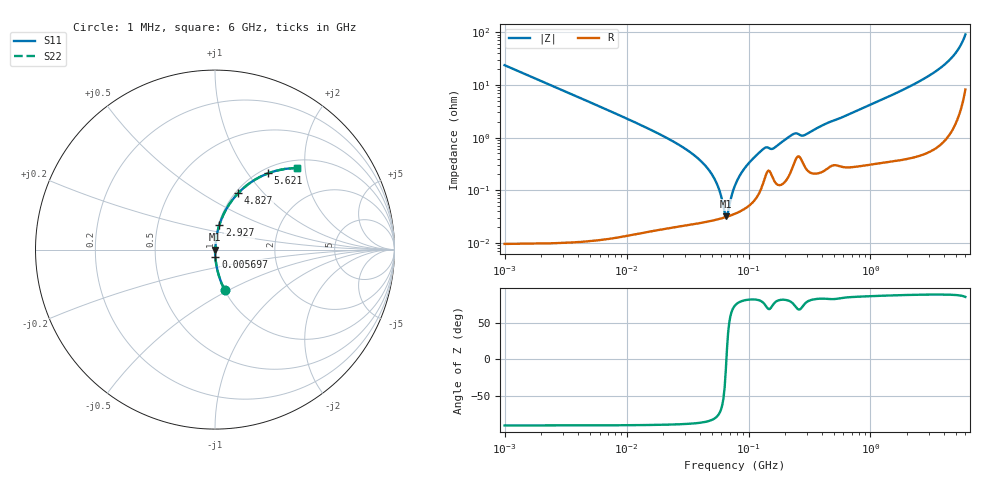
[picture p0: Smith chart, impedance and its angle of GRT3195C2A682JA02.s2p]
!Murata Part Number: GRT3195C2A682JA02
!These Parameters are Measured in Series Mode Connection
!Data Generated on Jun 19, 2026
!  o--ll--o
!Port1  Port2
!  o------o
!Operation Temp=25[degC], DC Bias Voltage=0[V]
!Freq. Start=1000[kHz] Stop=6[GHz] 401[Steps]
# Hz S RI R 50
!Freq.(Hz) S11(Real) S11(Imag) S21(Real) S21(Imag) S12(Real) S12(Imag) S22(Real) S22(Imag)
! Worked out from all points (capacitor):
!   401 points, 1 MHz to 6 GHz, reference 50 ohm
!   read as one part in series: C = 6.73 nF near 1.044 MHz
!   lowest |Z| = 32.2 mohm at 65.09 MHz (marker M1)
!   series resonance near 65.87 MHz, so ESL is about 870 pH
!   S11 on the Smith chart (normalised r, x): 1 MHz: 1.00, -0.47; 5.697 MHz: 1.00, -0.08; 2.927 GHz: 1.01, +0.29; 4.827 GHz: 1.03, +0.73; 5.621 GHz: 1.08, +1.25; 6 GHz: 1.16, +1.80
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1000000  0.053 -0.2238  0.947 0.2238  0.947 0.2238  0.053 -0.2238
4293785  0.0031 -0.0546  0.9969 0.0546  0.9969 0.0546  0.0031 -0.0546
5696791  0.0018 -0.0411  0.9982 0.0411  0.9982 0.0411  0.0018 -0.0411
1.843659e7  0.000316 -0.0118  0.9997 0.0118  0.9997 0.0118  0.000316 -0.0118
3.175522e7  0.000251 -0.00569  0.9997 0.00569  0.9997 0.00569  0.000251 -0.00569
4.497189e7  0.000259 -0.0028  0.9997 0.0028  0.9997 0.0028  0.000259 -0.0028
5.469524e7  0.00028 -0.00134  0.9997 0.00134  0.9997 0.00134  0.00028 -0.00134
6.508975e7  0.000311 -8.51e-05  0.9997 8.51e-05  0.9997 8.51e-05  0.000311 -8.51e-05
6.798347e7  0.000321 0.000229  0.9997 -0.000229  0.9997 -0.000229  0.000321 0.000229
7.745967e7  0.000361 0.00118  0.9996 -0.00118  0.9996 -0.00118  0.000361 0.00118
8.450008e7  0.000398 0.00184  0.9996 -0.00184  0.9996 -0.00184  0.000398 0.00184
9.420718e7  0.000462 0.0027  0.9995 -0.0027  0.9995 -0.0027  0.000462 0.0027
1.334167e8  0.00151 0.00599  0.9985 -0.00599  0.9985 -0.00599  0.00151 0.00599
1.622626e8  0.00156 0.00616  0.9984 -0.00616  0.9984 -0.00616  0.00156 0.00616
2.348496e8  0.00323 0.0113  0.9968 -0.0113  0.9968 -0.0113  0.00323 0.0113
2.794814e8  0.00339 0.0103  0.9966 -0.0103  0.9966 -0.0103  0.00339 0.0103
3.325952e8  0.00227 0.0133  0.9977 -0.0133  0.9977 -0.0133  0.00227 0.0133
1.428092e9  0.00709 0.0602  0.9929 -0.0602  0.9929 -0.0602  0.00709 0.0602
2.927209e9  0.0248 0.1386  0.9752 -0.1386  0.9752 -0.1386  0.0248 0.1386
4.827224e9  0.1281 0.3135  0.8719 -0.3135  0.8719 -0.3135  0.1281 0.3135
5.62102e9  0.2951 0.4248  0.7049 -0.4248  0.7049 -0.4248  0.2951 0.4248
6e9  0.4541 0.4546  0.5459 -0.4546  0.5459 -0.4546  0.4541 0.4546
